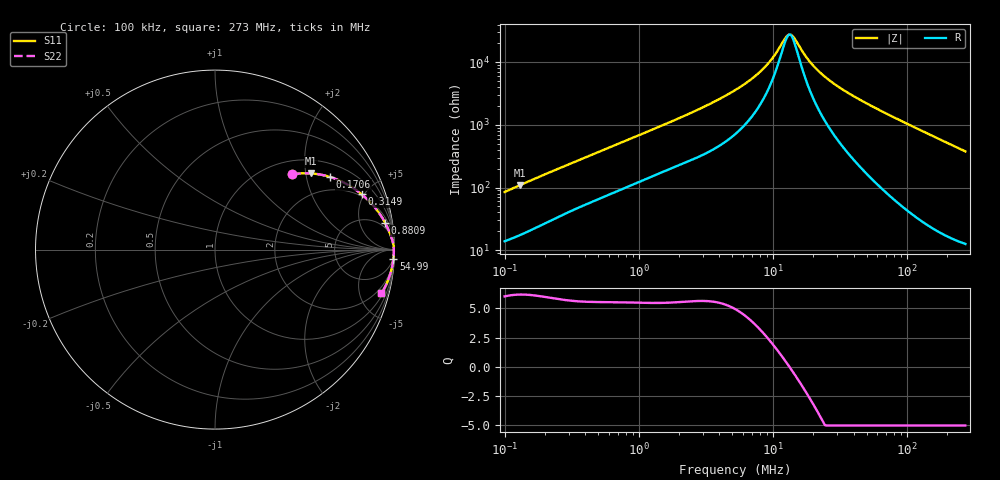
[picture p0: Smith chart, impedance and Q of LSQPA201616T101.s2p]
! LSQPA201616T101  S-PARAMETER MODEL  ( General Type )
! Model Generated by TAIYO YUDEN Corporation (http://www.ty-top.com)
! Version 2.0
! TAIYO YUDEN Control No. 100810NF25SB-FKC
! Copyright(c) 2007 TAIYO YUDEN CO.,LTD. All Rights Reserved.
! Product Description (link to TY-COMPAS)
! https://ds.yuden.co.jp/TYCOMPAS/or/detail?pn=LSQPA201616T101K&u=M
! Products Name : Inductors
! Characteristics :
!  Inductance : 100 uH , SRF(min) : 8.0 MHz , DC Resistance(max) : 10.4 Ohm
!  Rated Current : Saturation :110 mA , Temp Rise : 110 mA (40 degC)
!  Case Size : 2.0 x 1.6 / 0.079 x 0.063 [mm/inch] , Thickness : 1.6 / 0.063 [mm/inch]
!  (Conditions: Temperature = 25 degC , DC Bias Current/Voltage = 0A / 0V)
! External Node Assignments :
!  1  o---GGG---o  2
! GND o---------o GND
! Frequency Range : 0.1MHz  -  272.98108MHz  [ 402 STEP ]
# MHz S RI R 50
! Freq[MHz].  S11 Real  S11 Imag  S21 Real  S21 Imag  S12 Real  S12 Imag  S22 Real  S22 Imag
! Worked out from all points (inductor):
!   401 points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, 100 kHz to 273 MHz, reference 50 ohm
!   read as one part in series: L = 132 uH near 104 kHz
!   highest Q = 6.19 at 129.3 kHz (marker M1), where L = 132 uH
!   self-resonance near 13.24 MHz
!   S11 on the Smith chart (normalised r, x): 100 kHz: 1.28, +1.67; 170.6 kHz: 1.45, +2.77; 314.9 kHz: 1.85, +4.81; 880.9 kHz: 3, +12; 54.99 MHz: 4, -40; 273 MHz: 1.25, -7.54
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0.1  0.43 0.4191  0.57 -0.4191  0.57 -0.4191  0.43 0.4191
0.129323  0.5347 0.4245  0.4653 -0.4245  0.4653 -0.4245  0.5347 0.4245
0.170584  0.6418 0.4045  0.3582 -0.4045  0.3582 -0.4045  0.6418 0.4045
0.314948  0.8175 0.3078  0.1825 -0.3078  0.1825 -0.3078  0.8175 0.3078
0.376316  0.8522 0.2766  0.1478 -0.2766  0.1478 -0.2766  0.8522 0.2766
0.88092  0.9481 0.149  0.0519 -0.149  0.0519 -0.149  0.9481 0.149
1.416134  0.9706 0.1006  0.0294 -0.1006  0.0294 -0.1006  0.9706 0.1006
3.062861  0.9886 0.0497  0.0114 -0.0497  0.0114 -0.0497  0.9886 0.0497
5.329134  0.9939 0.0264  0.00612 -0.0264  0.00612 -0.0264  0.9939 0.0264
6.891772  0.9951 0.018  0.0049 -0.018  0.0049 -0.018  0.9951 0.018
8.566917  0.9958 0.0117  0.00424 -0.0117  0.00424 -0.0117  0.9958 0.0117
10.23617  0.9961 0.00684  0.00389 -0.00684  0.00389 -0.00684  0.9961 0.00684
12.47501  0.9964 0.0017  0.00364 -0.0017  0.00364 -0.0017  0.9964 0.0017
13.23768  0.9964 0.00018  0.00359 -0.00018  0.00359 -0.00018  0.9964 0.00018
14.32759  0.9965 -0.00185  0.00354 0.00185  0.00354 0.00185  0.9965 -0.00185
17.11931  0.9965 -0.0065  0.00349 0.0065  0.00349 0.0065  0.9965 -0.0065
19.66158  0.9965 -0.0103  0.0035 0.0103  0.0035 0.0103  0.9965 -0.0103
29.20284  0.9962 -0.0223  0.00383 0.0223  0.00383 0.0223  0.9962 -0.0223
54.99405  0.9941 -0.0499  0.00594 0.0499  0.00594 0.0499  0.9941 -0.0499
73.9896  0.9916 -0.0688  0.00839 0.0688  0.00839 0.0688  0.9916 -0.0688
144.9579  0.9763 -0.1359  0.0237 0.1359  0.0237 0.1359  0.9763 -0.1359
272.9811  0.9273 -0.2435  0.0727 0.2435  0.0727 0.2435  0.9273 -0.2435
